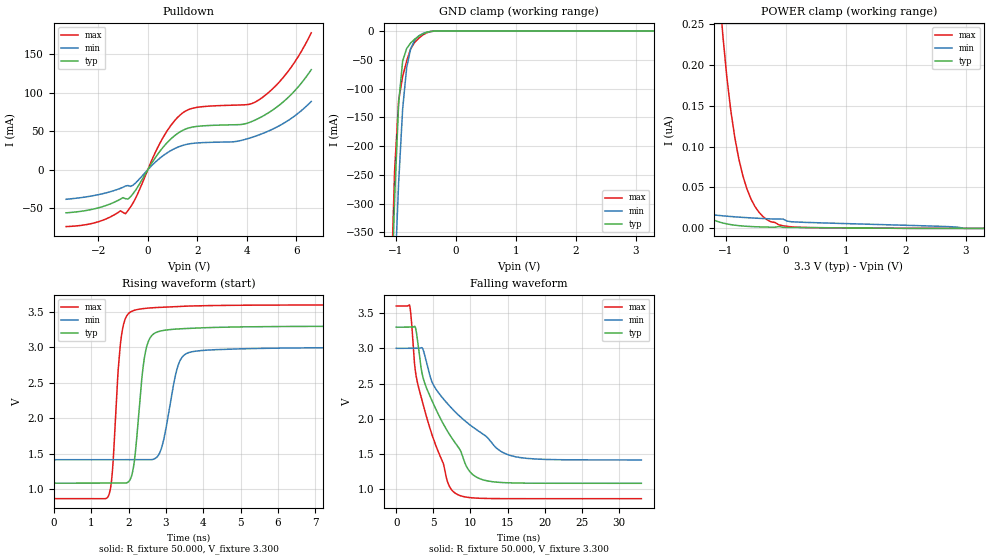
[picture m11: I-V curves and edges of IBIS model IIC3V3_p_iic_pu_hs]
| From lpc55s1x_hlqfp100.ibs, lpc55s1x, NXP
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|   Model IIC3V3_p_iic_pu_hs
[Model] IIC3V3_p_iic_pu_hs
Model_type I/O_open_drain
Polarity   Non-Inverting
Enable   Active-Low
Vinl =  0.990V
Vinh =  2.310V
Vmeas =  1.650V
Cref =  0.0F
Rref =  100.000
Vref =  3.3V
C_comp   2.434pF   2.433pF   2.440pF
C_comp_pulldown   1.614pF   1.554pF   1.665pF
C_comp_power_clamp   0.538pF   0.436pF   0.627pF
[Model Spec]
Vinh   2.310V   2.100V   2.520V
Vinl   0.990V   0.900V   1.080V
Vmeas   1.650V   1.500V   1.800V
Vref   3.3V   3.0V   3.6V
Cref   0.0F   0.0F   0.0F
Rref   100.000   100.000   100.000
[Temperature Range]   25.000   0.125k   -40.000
[Voltage Range]   3.300V   3.000V   3.600V
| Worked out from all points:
|   slope of the pulldown table from 0 to 0.495 V, typ, clamps not added: 20.4 ohm
|   GND clamp passes 1 mA (typ) near -0.43 V on its own axis
|   rising waveform, R_fixture 50.000, V_fixture 3.300: 20-80 % time 241ps typ, 336ps min, 194ps max; typ from 1.08 V to 3.3 V
|   falling waveform, R_fixture 50.000, V_fixture 3.300: 20-80 % time 5.55ns typ, 7.92ns min, 3.88ns max; typ from 3.3 V to 1.08 V
[Pulldown]
|Voltage   I(typ)   I(min)   I(max)
-3.3V     -56mA      -38.4mA    -73.87mA
-2.1V     -50.37mA   -33.07mA   -68.52mA
-1.1V     -38.15mA   -24.11mA   -53.37mA
-900mV    -37.61mA   -21.16mA   -57.18mA
-500mV    -26.92mA   -17.4mA    -37.43mA
500mV     24.51mA    15.34mA    35.14mA
1.2V      47.07mA    29.16mA    67.89mA
1.9V      55.94mA    34.55mA    80.54mA
3.8V      58.93mA    38.31mA    84.23mA
4.5V      67.16mA    45.4mA     91.05mA
5.6V      91.88mA    62.62mA    125.1mA
6.6V      130mA      88.76mA    177.9mA
[GND_clamp]
|Voltage   I(typ)   I(min)   I(max)
-3.3V     -10.05A    -9.18A     -11.33A
-1.089V   -516.5mA   -633.7mA   -475mA
-1.022V   -291.8mA   -436.3mA   -243.2mA
-955mV    -126mA     -264mA     -120.7mA
-888mV    -52.17mA   -135.6mA   -79.11mA
-821mV    -30.43mA   -63.68mA   -52.11mA
-754mV    -20.66mA   -30.68mA   -31.04mA
-687mV    -14.18mA   -15.96mA   -19.64mA
-553mV    -5.013mA   -4.505mA   -7.034mA
-419mV    -652.2uA   -708.2uA   -887.6uA
-285mV    -14.83uA   -32.68uA   -16.3uA
3.3V      0A         0A         0A
[POWER_clamp]
|Voltage   I(typ)   I(min)   I(max)
-3.3V     1.337uA    96.84nA    41.74uA
-2.395V   241.1nA    38.51nA    8.841uA
-2.194V   152.2nA    32.17nA    5.805uA
-1.926V   78.16nA    25.86nA    3.134uA
-1.658V   37.82nA    21.36nA    1.572uA
-1.256V   11.75nA    16.9nA     472.7nA
-1.055V   6.592nA    15.36nA    237.1nA
-921mV    4.605nA    14.51nA    144.1nA
-787mV    3.339nA    13.77nA    84.89nA
-586mV    2.257nA    12.84nA    36.19nA
-318mV    1.588nA    11.83nA    10.67nA
3.3V      0A         0A         0A
[Ramp]
| variable   typ   min   max
dV/dt_r   1.329/0.241n   0.950/0.336n   1.640/0.194n
dV/dt_f   1.329/5.554n   0.950/7.920n   1.640/3.875n
R_load = 50.000
[Rising Waveform]
R_fixture= 50.000
V_fixture= 3.300
V_fixture_min= 3.000
V_fixture_max= 3.600
|time   V(typ)   V(min)   V(max)
0s        1.085V     1.416V     866.9mV
1.467ns   1.085V     1.416V     908.8mV
1.83ns    1.085V     1.416V     3.231V
2.114ns   1.255V     1.416V     3.516V
2.303ns   2.25V      1.416V     3.542V
2.618ns   3.165V     1.417V     3.559V
2.901ns   3.237V     1.61V      3.568V
3.354ns   3.262V     2.784V     3.58V
3.886ns   3.275V     2.953V     3.588V
33ns      3.3V       3V         3.6V
[Falling Waveform]
R_fixture= 50.000
V_fixture= 3.300
V_fixture_min= 3.000
V_fixture_max= 3.600
|time   V(typ)   V(min)   V(max)
0s        3.3V       3V         3.6V
1.816ns   3.3V       3V         3.608V
2.49ns    3.313V     3V         2.758V
2.916ns   3.083V     3V         2.487V
3.929ns   2.479V     2.866V     2.084V
5.006ns   2.213V     2.482V     1.717V
7.803ns   1.679V     2.113V     955.9mV
12.03ns   1.125V     1.757V     870.3mV
16.66ns   1.088V     1.451V     867.2mV
33ns      1.085V     1.416V     866.9mV
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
